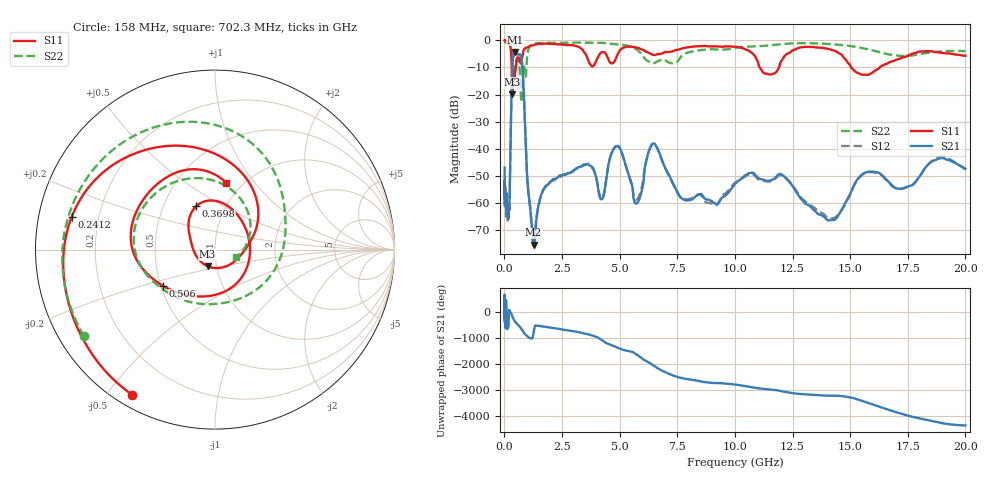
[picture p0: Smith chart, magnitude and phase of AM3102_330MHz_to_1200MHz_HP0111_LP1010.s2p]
! Date/Time: Tue, Sep 11, 2018 5:16 PM
! Network Analyzer: Agilent Technologies E8362B Rev: A.07.50.63
! Sweep from 0.010 to 20.000 GHz, 1601 Points, Sweep Type: LOG
! Power Supply: 4.949 V, 0.001 A
# Hz S DB R 50
!freq MagS11 AngS11 MagS21 AngS21 MagS12 AngS12 MagS22 AngS22
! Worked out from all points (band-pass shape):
!   1601 points, 10 MHz to 20 GHz, reference 50 ohm
!   highest |S21| = -4.22 dB at 478 MHz (marker M1); lowest = -75.6 dB at 1.266 GHz (marker M2)
!   |S21| within 3 dB of the highest: 362.9 MHz to 752.1 MHz (389.2 MHz wide, 69.8 % of centre)
!   lowest |S11| = -19.9 dB at 341.1 MHz (marker M3), VSWR 1.23, Z = 45.3 - j8.46 ohm
!   |S11| at or under -10 dB: 317.4 MHz to 495.5 MHz (178.1 MHz wide, 43.8 % of centre); 11.08 GHz to 11.91 GHz (832.2 MHz wide, 7.24 % of centre); 15.04 GHz to 16.28 GHz (1.239 GHz wide, 7.91 % of centre)
!   |S22| runs from -22.9 to -0.3 dB; largest |S21 - S12| = 0.011
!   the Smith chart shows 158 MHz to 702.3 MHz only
!   S11 on the Smith chart (normalised r, x): 158 MHz: 0.05, -0.58; 241.2 MHz: 0.10, +0.11; 369.8 MHz: 0.73, +0.38; 506 MHz: 0.51, -0.24; 702.3 MHz: 0.84, +0.73
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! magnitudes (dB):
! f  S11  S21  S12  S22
! 10 MHz  0.0  -47.1  -53.2  -0.3
! 35.55 MHz  0.0  -58.5  -58.3  -0.5
! 126.4 MHz  -0.4  -62.8  -61.1  -1.0
! 158 MHz  -0.6  -64.9  -65.3  -1.2
! 241.2 MHz  -1.7  -51.4  -51.7  -1.8
! 341.1 MHz  -19.9  -9.9  -9.9  -6.5
! 369.8 MHz  -11.6  -6.7  -6.8  -8.6
! 447.2 MHz  -13.4  -4.3  -4.4  -9.9
! 478 MHz  -11.5  -4.2  -4.2  -9.0
! 506 MHz  -9.0  -4.3  -4.5  -7.9
! 702.3 MHz  -8.5  -5.4  -5.4  -18.2
! 1.266 GHz  -1.7  -75.6  -75.8  -1.3
! 1.59 GHz  -1.3  -57.3  -57.5  -0.9
! 3.599 GHz  -6.5  -45.8  -45.7  -0.8
! 4.23 GHz  -4.3  -58.7  -58.8  -0.9
! 4.878 GHz  -5.9  -39.1  -39.1  -1.5
! 5.652 GHz  -2.4  -59.9  -58.5  -2.9
! 6.457 GHz  -5.3  -38.1  -38.3  -8.4
! 7.808 GHz  -2.8  -58.9  -58.8  -5.0
! 11.92 GHz  -9.9  -49.5  -49.9  -1.5
! 14.01 GHz  -3.1  -66.4  -65.5  -1.3
! 20 GHz  -5.6  -47.4  -47.7  -3.9
